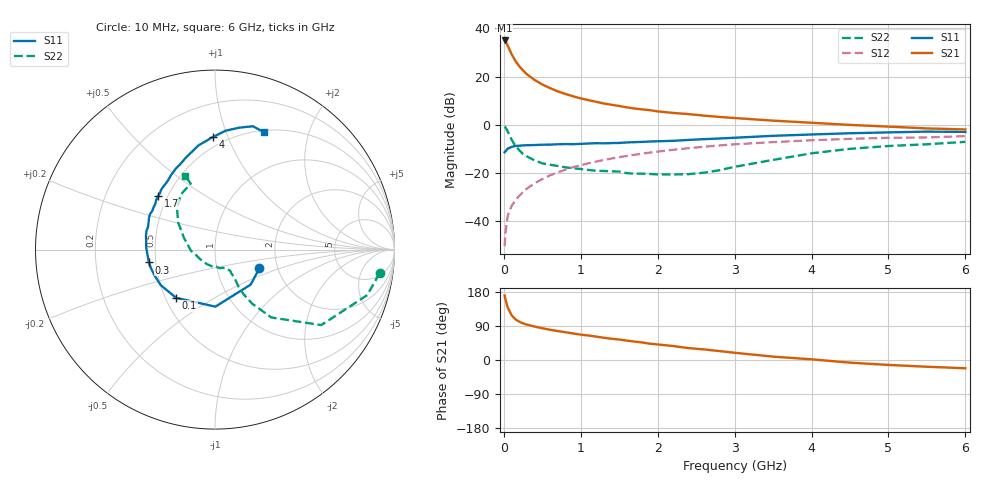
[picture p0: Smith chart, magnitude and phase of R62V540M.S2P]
! SIEMENS Small Signal Semiconductors
! BFR193
! Si NPN RF Bipolar Junction Transistor in SOT23
! VCE = 2.5 V  IC = 40 mA
! Common Emitter S-Parameters:  May  1996
# GHz  S  MA  R  50
!  f  S11  S21  S12  S22
! GHz  MAG  ANG  MAG  ANG  MAG  ANG  MAG  ANG
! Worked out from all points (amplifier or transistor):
!   36 points, 10 MHz to 6 GHz, reference 50 ohm
!   highest |S21| = 35.0 dB at 10 MHz (marker M1)
!   |S21| within 3 dB of that: start of sweep to 62.38 MHz
!   unconditionally stable (mu >= 1): 393.1 MHz to 1.869 GHz; 1.968 GHz to 2.034 GHz
!   at 250 MHz: K = 0.95, MSG = 25.2 dB, |S12| = -28.0 dB
!   at 1.4 GHz: K = 1.02, MAG = 10.3 dB, |S12| = -14.0 dB
!   at 6 GHz: K = 0.95, MSG = 1.4 dB, |S12| = -4.7 dB
!   S11 on the Smith chart (normalised r, x): 10 MHz: 1.61, -0.36; 100 MHz: 0.57, -0.35; 300 MHz: 0.46, -0.08; 1.7 GHz: 0.45, +0.33; 4 GHz: 0.43, +0.88; 6 GHz: 0.52, +1.37
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0.01  0.2685 -23.0  56.26 170.1  0.003 79.5  0.9262 -8.2
0.02  0.2785 -44.5  54.23 160.6  0.0055 80.3  0.8857 -16.6
0.05  0.3179 -89.6  44.02 138.6  0.0128 71.5  0.7262 -35.4
0.1  0.3452 -128.9  29.39 118.3  0.0205 68.0  0.4914 -50.3
0.15  0.3611 -146.5  21.2 107.5  0.0268 68.4  0.3649 -55.5
0.2  0.3664 -156.9  16.45 101.1  0.0333 70.7  0.2955 -57.3
0.25  0.3715 -164.0  13.34 96.5  0.04 71.7  0.246 -57.6
0.3  0.3748 -169.0  11.2 93.4  0.0472 72.6  0.2194 -56.7
0.4  0.3782 -176.8  8.524 88.2  0.0607 73.3  0.1818 -55.3
0.5  0.3842 177.9  6.845 83.8  0.0745 73.7  0.1578 -55.4
0.6  0.3859 173.2  5.757 79.8  0.0888 72.9  0.1476 -54.4
0.7  0.3923 168.7  4.943 76.4  0.1024 72.2  0.139 -55.5
0.8  0.3959 164.8  4.361 73.3  0.1166 71.0  0.1304 -58.0
1.1  0.4073 154.7  3.24 64.6  0.1579 67.6  0.1148 -63.8
1.3  0.4106 148.5  2.757 58.7  0.1855 64.8  0.1094 -68.9
1.7  0.4347 136.7  2.167 48.6  0.238 59.1  0.096 -85.5
2.2  0.4626 125.2  1.759 36.9  0.3014 51.5  0.0927 -118.2
3.5  0.5879 99.0  1.215 8.9  0.4355 30.9  0.1858 158.9
4  0.6266 91.2  1.098 1.8  0.4747 23.7  0.2547 143.7
4.5  0.665 84.9  0.991 -7.0  0.509 16.7  0.3155 132.2
5.5  0.719 72.9  0.838 -17.8  0.5443 2.8  0.3921 110.2
6  0.7086 67.3  0.797 -21.8  0.5791 -1.3  0.4412 112.0
